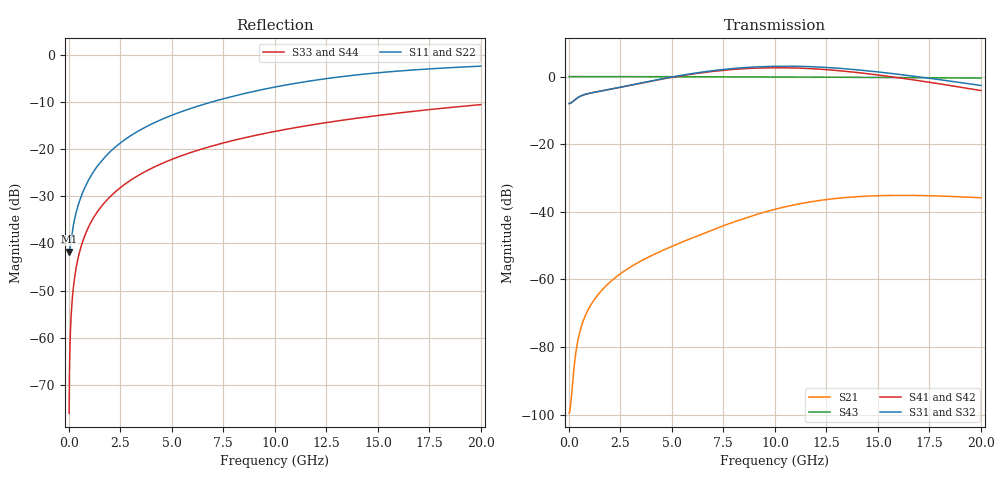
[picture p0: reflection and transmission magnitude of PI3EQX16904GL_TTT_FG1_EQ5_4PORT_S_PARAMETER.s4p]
! NPort=4 DATA=2000 NOISE=0 GROUPDELAY=0 COMPLEX_DATAFORMAT=POLAR
! NumOfBlock=1 NumOfParam=0
! .MODEL Smodel S TSTONEFILE=PI3EQX16904GL_TTT_FG1_EQ5_4PORT_S_PARAMETER.s4p TYPE=S
!  -- The above .MODEL line can be used for the S element in the netlist.
! The s parameter is extracted from the linear redriver, it is not bi-directional; only s(4,1)s(4,2) and s(3,1)s(3,2)
! should be the insertion loss
!Port definition:
!Port1 = input+
!Port2 = input-
!Port3 = output+
!Port4 = output-
# Hz S MA R  50
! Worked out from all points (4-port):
!   2000 points, 10 MHz to 20 GHz, reference 50 ohm
!   strongest paths, dB at 10 MHz, 5.01 GHz, 10.01 GHz, 15.01 GHz, 20 GHz:
!     S31: -8.0, -0.1, 3.1, 1.4, -2.6
!     S32: -8.0, -0.2, 2.9, 1.2, -2.8
!     S41: -8.0, -0.2, 2.6, 0.5, -4.1
!     S42: -8.0, -0.4, 2.4, 0.3, -4.3
!     S43: 0.0, 0.0, -0.1, -0.3, -0.4
!     S21: -99.6, -50.2, -39.2, -35.2, -35.8
!   lowest |S11| = -41.7 dB at 10 MHz (marker M1), VSWR 1.02, Z = 49.2 - j0.0603 ohm
!   |S11| at or under -10 dB: start of sweep to 6.888 GHz
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1e7  0.008182 -175.7  1.05e-05 7.7  0 0.0  0 0.0
     1.05e-05 7.7  0.008182 -175.7  0 0.0  0 0.0
     0.3996 0.5  0.3996 -179.5  0.0001571 -90.0  1 -0.0
     0.3996 -179.6  0.3996 0.4  1 -0.0  0.0001571 -90.0
3.9e8  0.02299 -119.3  0.0001056 117.8  0 0.0  0 0.0
       0.0001056 117.8  0.02299 -119.3  0 0.0  0 0.0
       0.4799 10.4  0.4797 -169.7  0.006126 -90.4  1 -0.4
       0.4799 -170.3  0.4796 9.6  1 -0.4  0.006126 -90.4
1.63e9  0.07746 -102.7  0.0007112 107.3  0 0.0  0 0.0
        0.000711 107.3  0.07746 -102.7  0 0.0  0 0.0
        0.6186 3.8  0.6174 -176.6  0.02559 -91.5  0.9996 -1.5
        0.6178 -179.1  0.6166 0.5  0.9996 -1.5  0.02559 -91.5
6.01e9  0.2762 -104.9  0.004176 94.3  0 0.0  0 0.0
        0.004144 94.4  0.2761 -105.0  0 0.0  0 0.0
        1.112 -37.6  1.09 141.6  0.09395 -95.6  0.9952 -5.4
        1.092 131.7  1.071 -49.0  0.9952 -5.4  0.09395 -95.6
9.89e9  0.4537 -112.5  0.01078 65.8  0 0.0  0 0.0
        0.01069 66.6  0.4534 -112.5  0 0.0  0 0.0
        1.419 -97.8  1.387 81.8  0.1534 -99.2  0.9872 -8.8
        1.353 65.0  1.323 -115.5  0.9872 -8.8  0.1534 -99.2
1.402e10  0.6189 -123.0  0.01688 18.8  0 0.0  0 0.0
          0.01678 20.1  0.6186 -123.0  0 0.0  0 0.0
          1.257 -164.5  1.229 15.1  0.2147 -102.9  0.9748 -12.4
          1.146 -8.2  1.121 171.4  0.9748 -12.4  0.2147 -102.9
2e10  0.7644 -136.2  0.01617 -34.9  0 0.0  0 0.0
      0.01615 -33.0  0.7645 -136.1  0 0.0  0 0.0
      0.7386 114.9  0.7209 -65.5  0.2986 -108.1  0.9506 -17.4
      0.6219 -97.0  0.607 82.6  0.9506 -17.4  0.2986 -108.1
